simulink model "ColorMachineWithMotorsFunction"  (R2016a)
settings: Solver=FixedStepAuto  StartTime=0.0  StopTime=inf  RelTol=1e-3
libraries: miniQ x3

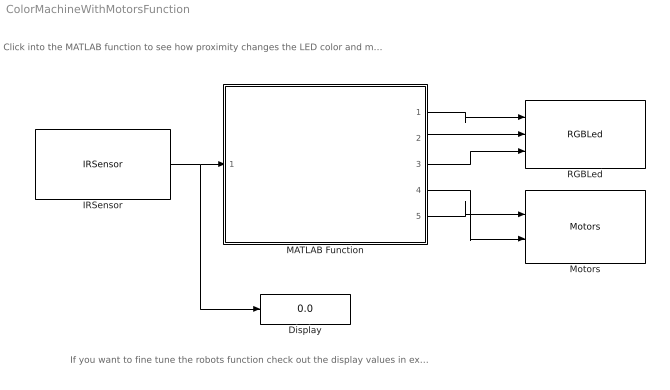
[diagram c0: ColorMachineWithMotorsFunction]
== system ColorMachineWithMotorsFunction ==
  note: If you want to fine tune the robots function check out the display values in external mode here.
  note: Click into the MATLAB function to see how proximity changes the LED color and motor directions respectively.
  Display : Display
  IRSensor : miniQ/IRSensor  sampleTime_dd=0.01  debug_dd=off
  MATLAB Function : MATLAB Function  TreatAsAtomicUnit=on
  Motors : miniQ/Motors  flipLeft=off  flipRight=off
  RGBLed : miniQ/RGBLed
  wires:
  IRSensor/1 -> Display/1, MATLAB Function/1(proximity)
  MATLAB Function/1(red) -> RGBLed/1
  MATLAB Function/2(green) -> RGBLed/2
  MATLAB Function/3(blue) -> RGBLed/3
  MATLAB Function/4(MR) -> Motors/2
  MATLAB Function/5(ML) -> Motors/1

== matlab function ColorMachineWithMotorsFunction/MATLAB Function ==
function [red,green,blue,MR,ML] = colormachineWithMotors(proximity)
if proximity <10
    red = 0;
    green=255;
    blue = 0;
    MR = 255;%Right motor
    ML = 255;%Left motor
elseif proximity >10 && proximity<20
    red=255;
    green=0;
    blue = 0;
    MR = 255;
    ML = -255;
else
    red=0;
    green=0;
    blue=255;
    MR = -255;
    ML = 255;
end
